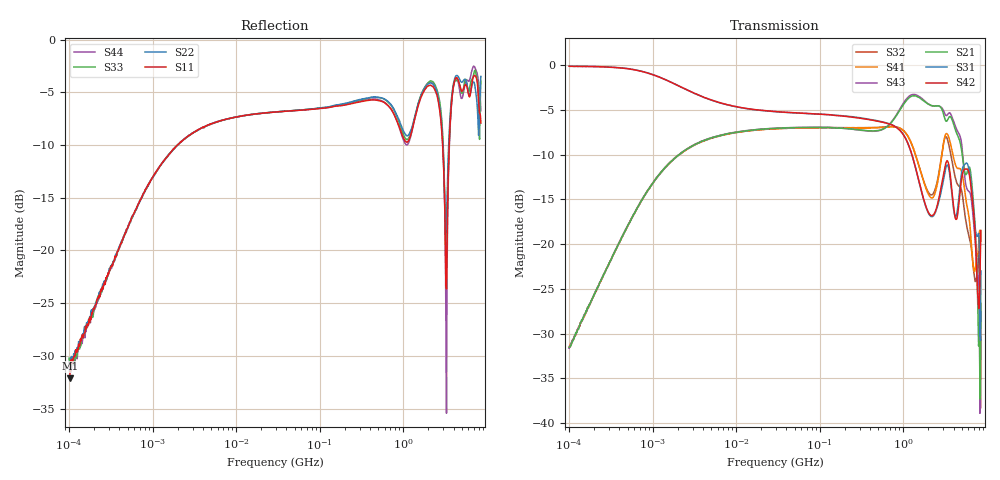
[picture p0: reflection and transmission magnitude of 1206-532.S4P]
!Agilent Technologies,E5071C,MY46110495,A.10.06
!Date: Tue Jun 06 11:47:29 2017
!Data & Calibration Information:
!Freq	S11:SOLT4(ON)	S12:SOLT4(ON)	S13:SOLT4(ON)	S14:SOLT4(ON)
!	S21:SOLT4(ON)	S22:SOLT4(ON)	S23:SOLT4(ON)	S24:SOLT4(ON)
!	S31:SOLT4(ON)	S32:SOLT4(ON)	S33:SOLT4(ON)	S34:SOLT4(ON)
!	S41:SOLT4(ON)	S42:SOLT4(ON)	S43:SOLT4(ON)	S44:SOLT4(ON)
!PortZ  Port1:50+j0  Port2:50+j0  Port3:50+j0  Port4:50+j0
!Above PortZ is port z conversion or system Z0 setting when saving the data.
!When reading, reference impedance value at option line is always used.
# Hz S dB R 50
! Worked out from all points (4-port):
!   801 points, 100 kHz to 8.5 GHz, reference 50 ohm
!   strongest paths, dB at 100 kHz, 1.721 MHz, 29.51 MHz, 502.3 MHz, 8.5 GHz:
!     S42: -0.1, -2.0, -5.2, -6.3, -18.5
!     S31: -0.1, -2.0, -5.2, -6.2, -23.0
!     S21: -31.5, -10.6, -7.1, -7.3, -26.6
!     S43: -31.6, -10.6, -7.0, -7.3, -27.5
!     S41: -31.5, -10.6, -7.1, -7.0, -19.7
!     S32: -31.6, -10.7, -7.1, -6.9, -30.4
!   lowest |S11| = -32.1 dB at 101.7 kHz (marker M1), VSWR 1.05, Z = 50.7 + j2.4 ohm
!   |S11| at or under -10 dB: start of sweep to 1.978 MHz; 2.963 GHz to 3.548 GHz (585.1 MHz wide, 18 % of centre)
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100000  -31.90 77.0  -31.51 86.1  -0.09 -1.3  -31.57 -94.3
        -31.52 85.5  -31.19 67.8  -31.58 -94.6  -0.12 -1.3
        -0.10 -1.3  -31.60 -95.5  -30.22 83.5  -31.53 85.7
        -31.49 -94.1  -0.10 -1.4  -31.64 86.2  -30.60 74.0
101665  -32.13 73.3  -31.31 85.8  -0.09 -1.4  -31.50 -93.1
        -31.52 86.2  -31.61 70.4  -31.58 -94.8  -0.12 -1.4
        -0.10 -1.4  -31.38 -94.5  -31.08 81.5  -31.35 86.3
        -31.36 -93.4  -0.10 -1.5  -31.46 85.6  -31.24 72.7
3005646  -8.85 29.4  -8.98 29.3  -3.04 -14.6  -9.00 -151.1
         -8.99 29.2  -8.88 29.0  -9.02 -151.1  -3.05 -14.5
         -3.04 -14.5  -9.04 -151.0  -8.87 29.3  -8.97 29.3
         -8.98 -151.1  -3.03 -14.5  -8.98 29.3  -8.86 29.1
1.337058e9  -7.88 63.4  -3.40 0.4  -10.72 -123.9  -9.41 56.1
            -3.40 0.5  -7.66 60.2  -9.44 59.5  -10.72 -123.8
            -10.73 -123.9  -9.45 59.5  -7.70 60.6  -3.27 -0.1
            -9.39 56.1  -10.72 -123.8  -3.25 -0.0  -7.85 65.5
5.161627e9  -4.80 -84.6  -10.45 -52.2  -11.38 41.3  -12.46 -99.6
            -10.47 -52.1  -3.97 -85.8  -14.82 -109.7  -12.00 38.7
            -11.39 41.4  -14.82 -109.6  -4.93 -82.9  -10.03 -64.9
            -12.46 -99.4  -11.99 38.7  -10.02 -64.9  -5.34 -77.0
6.842542e9  -3.61 20.7  -14.80 -71.7  -15.47 -29.6  -22.35 111.2
            -14.78 -71.5  -4.02 14.1  -22.24 73.4  -15.80 -33.2
            -15.49 -29.3  -22.22 73.5  -3.52 16.4  -16.81 -65.7
            -22.34 111.6  -15.78 -33.1  -16.79 -65.6  -2.57 17.9
8.5e9  -7.91 108.0  -26.55 52.4  -22.97 36.4  -19.69 43.9
       -26.59 52.8  -3.48 123.2  -30.51 116.3  -18.50 11.9
       -22.98 36.6  -30.43 116.1  -3.94 126.9  -27.56 47.8
       -19.68 44.2  -18.47 12.2  -27.51 48.2  -6.74 95.8
